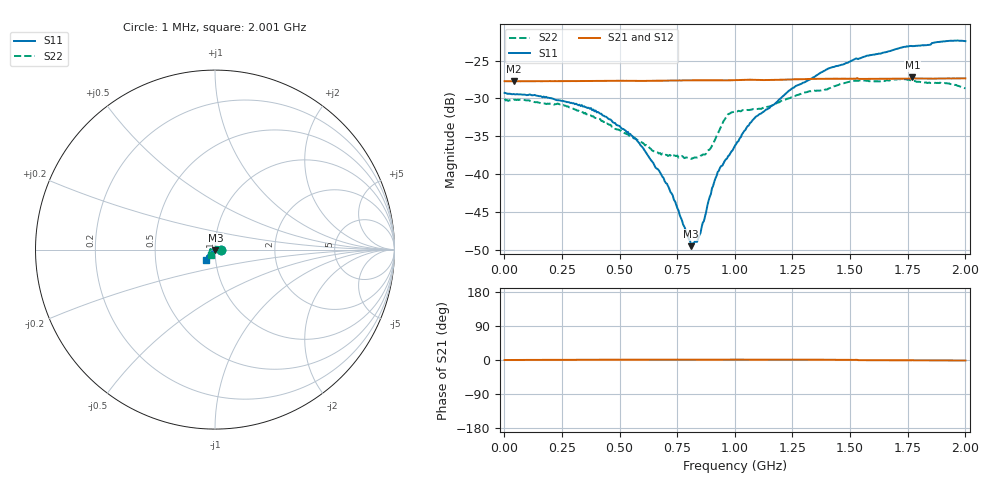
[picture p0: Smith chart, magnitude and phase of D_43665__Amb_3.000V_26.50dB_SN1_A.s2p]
! device id: 43665_
! dir: \\malibu\benchdata\1_engineers\tn_data\43665_75ohm\new\sparar\43665_\amb\3p000v\26p50db
! Serial: 1
! Insertion: A
! Temp: Amb
! VDD: 3.000V
! Attenuation Step: 26.50dB
! IDD: 1.448412e+00mA
! FILE NAME
! DATE 03-27-2009 08:39:53
! CORRECTED  DATA
#  Hz  S  RI  R  75
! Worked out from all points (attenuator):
!   401 points, 1 MHz to 2.001 GHz, reference 75 ohm
!   highest |S21| = -27.23 dB at 1.771 GHz (marker M1); lowest = -27.7 dB at 41 MHz (marker M2)
!   lowest |S11| = -49.5 dB at 811 MHz (marker M3), VSWR 1.01, Z = 75.3 - j0.428 ohm
!   |S11| at or under -10 dB: start of sweep to end of sweep
!   |S22| runs from -38.0 to -27.4 dB; largest |S21 - S12| = 0.00058
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1000000  0.0344 -0.000279  0.0411 -2.1e-05  0.0412 -3.27e-05  0.0315 -0.000111
4.1e7  0.0338 0.000512  0.0411 8.17e-05  0.0411 8.21e-06  0.031 0.00179
2.36e8  0.0307 0.00198  0.0412 0.000309  0.0412 0.000211  0.027 0.0107
3.36e8  0.0285 0.00218  0.0412 0.000393  0.0412 0.000258  0.0217 0.0139
4.16e8  0.0249 0.00262  0.0413 0.000546  0.0413 0.000373  0.0175 0.0152
5.46e8  0.0184 0.00168  0.0414 0.000517  0.0413 0.000312  0.00886 0.0155
6.71e8  0.0106 -0.000207  0.0415 0.000702  0.0414 0.000489  0.000605 0.0137
7.21e8  0.00752 -0.00113  0.0415 0.000742  0.0415 0.000501  -0.0024 0.0131
8.11e8  0.00177 -0.00285  0.0416 0.000653  0.0416 0.000402  -0.00907 0.00882
8.31e8  0.000646 -0.00353  0.0417 0.000658  0.0416 0.000393  -0.0105 0.00755
8.46e8  -0.000601 -0.0039  0.0417 0.000632  0.0416 0.00038  -0.0114 0.00645
8.86e8  -0.00405 -0.00529  0.0417 0.000582  0.0416 0.000318  -0.0141 0.00319
9.26e8  -0.00716 -0.00748  0.0416 0.000556  0.0416 0.000293  -0.0184 0.000216
9.66e8  -0.00924 -0.00868  0.0416 0.00073  0.0415 0.000444  -0.0242 0.000893
1.001e9  -0.0123 -0.0094  0.0418 0.000818  0.0417 0.00054  -0.0259 0.00196
1.096e9  -0.02 -0.0136  0.0419 0.00051  0.0419 0.000175  -0.0269 -0.00262
1.241e9  -0.0295 -0.0206  0.0422 0.000765  0.0422 0.000414  -0.0298 -0.0112
1.336e9  -0.0343 -0.026  0.0426 0.000615  0.0425 0.000253  -0.0316 -0.0161
1.521e9  -0.044 -0.037  0.0428 0.000246  0.0427 -0.000193  -0.0328 -0.0253
1.671e9  -0.0474 -0.0443  0.0427 -0.000501  0.0428 -0.000397  -0.0306 -0.0281
1.771e9  -0.0455 -0.0533  0.0435 -0.00043  0.043 -0.000616  -0.0278 -0.0306
2.001e9  -0.0495 -0.0571  0.0429 -0.00091  0.043 -0.000816  -0.0228 -0.029
